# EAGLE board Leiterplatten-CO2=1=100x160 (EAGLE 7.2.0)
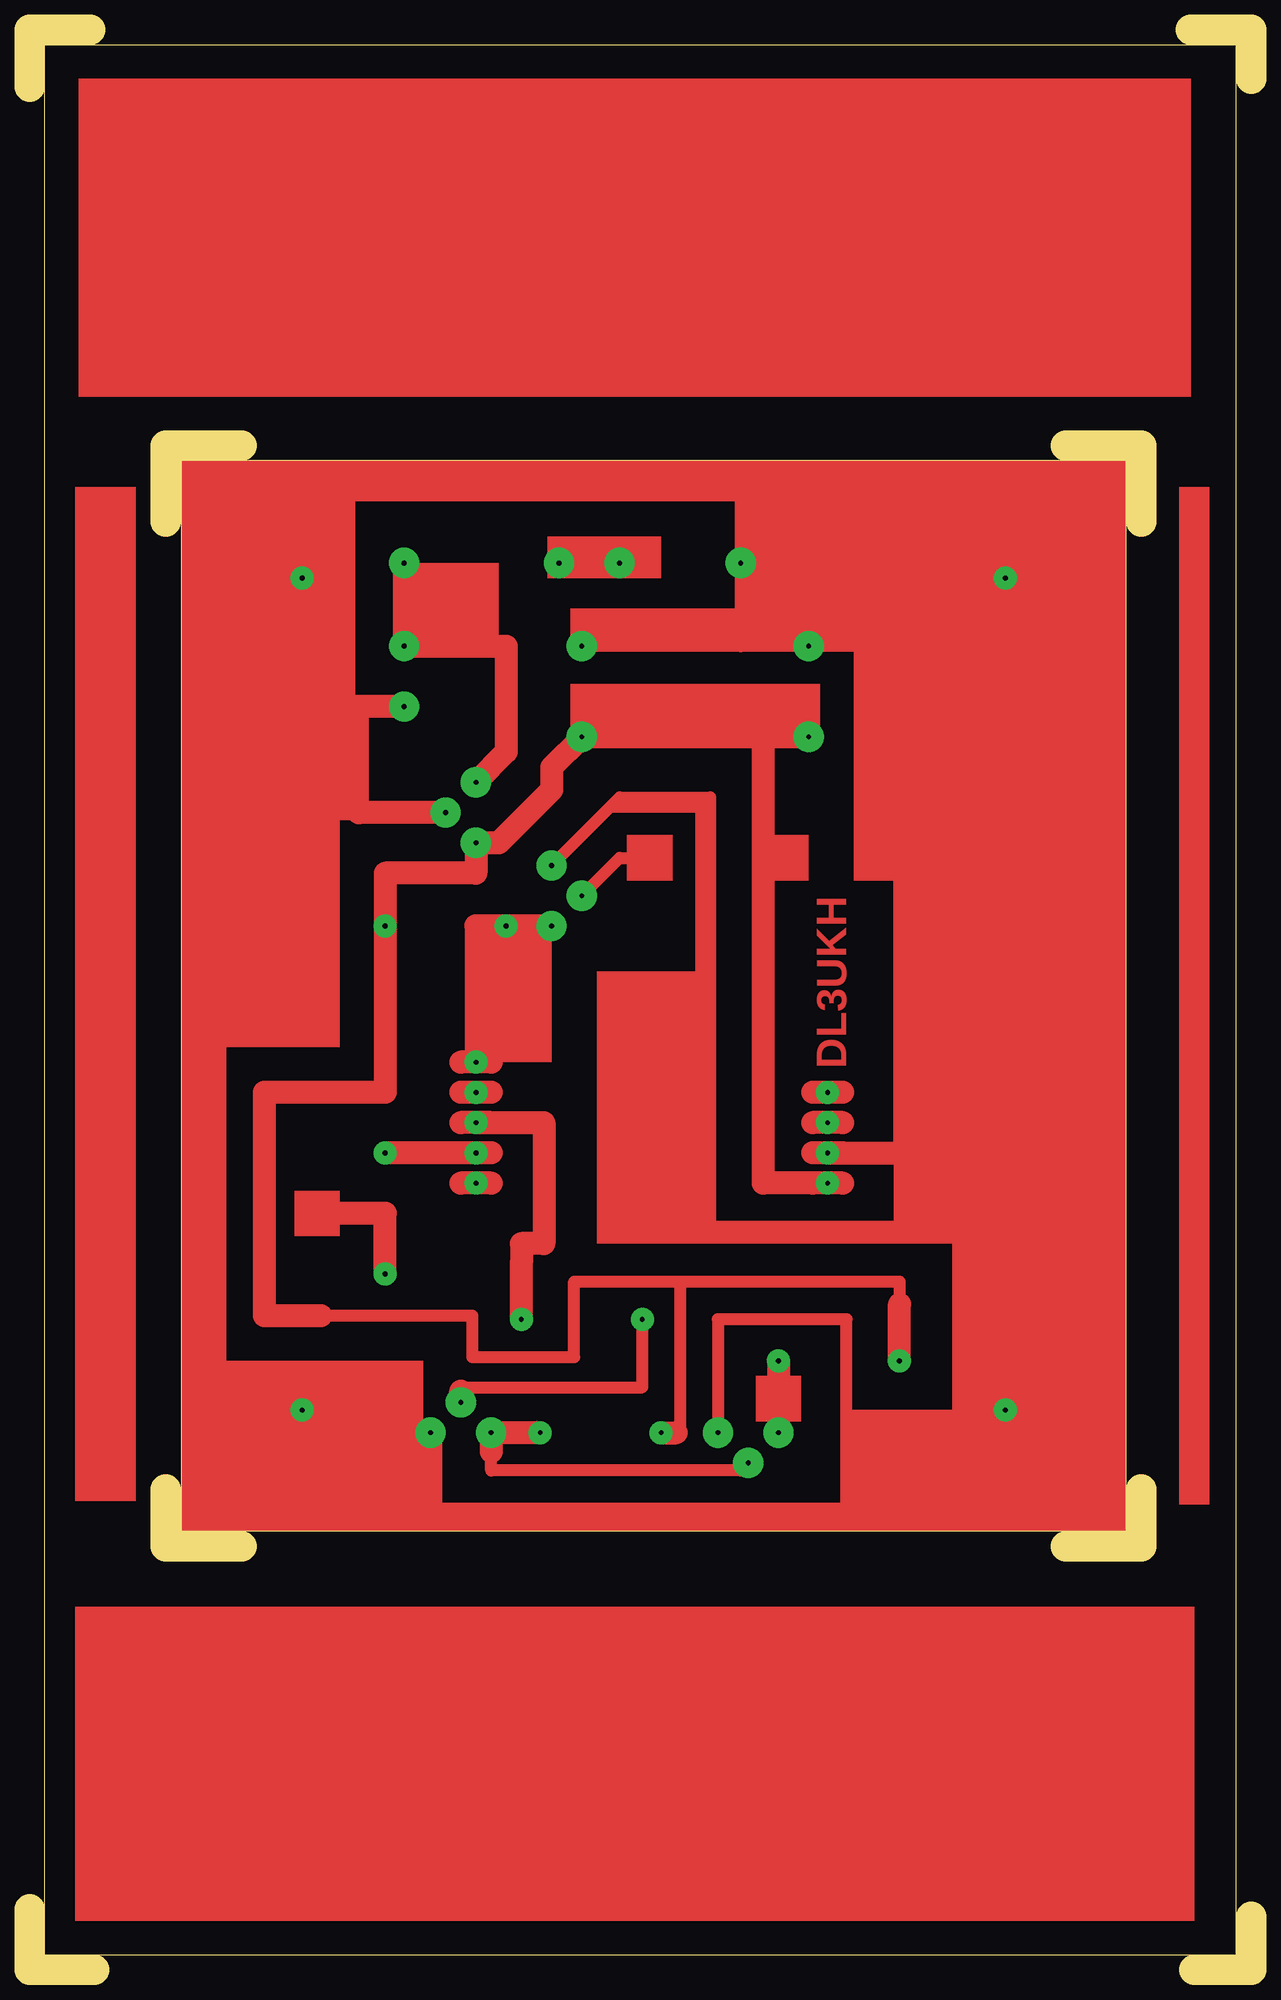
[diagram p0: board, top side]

Size 102.55 x 162.88 mm. Coordinates in mm from the lower left corner, seen from the top.
Outline: 5.4,0 0.32,0
Outline: 0,0 0,5.08
Outline: 97.79,0 102.55,0 102.55,4.45
Outline: 5.08,162.88 0,162.88 0,158.12
Outline: 102.55,158.75 102.55,162.88
Outline: 97.47,162.88 102.23,162.88
Outline: 11.43,121.6 11.43,127.95 17.78,127.95
Outline: 11.43,40.32 11.43,35.56 17.78,35.56
Outline: 86.99,35.56 93.34,35.56 93.34,40.32
Outline: 93.34,121.6 93.34,127.95 86.99,127.95
Outline: 1.27,1.27 101.28,1.27 101.28,161.61 1.27,161.61 1.27,1.27
Outline: 12.7,126.68 12.7,36.83 92.08,36.83 92.08,126.68 12.7,126.68
Copper layers (1*16): Top 0.035mm / dielectric 1.5mm / Bottom 0.035mm
Design rules "default": minimum track width 10mil, minimum drill 24mil, track to track 8mil, track to pad 8mil, pad to pad 8mil, via to via 8mil, smd to smd 8mil, copper to edge 40mil, drill to drill 8mil, minimum pad ring 10mil, minimum via ring 8mil, stop-mask expansion 4mil, vias tented up to drill 0mil, thermal gap 10mil

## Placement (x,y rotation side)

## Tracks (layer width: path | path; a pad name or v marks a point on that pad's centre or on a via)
S$1  (via drill 0.4 pad 1.93)
  Top 1.016: 37.47,71.12 37.15,71.12
  Top 1.93: 37.47,71.12 43.18,71.12 43.18,60.96 41.28,60.96 41.28,59.37 41.28,58.74 v41.28,54.61
S$2  (via drill 0.4 pad 1.93, 0.4 pad 2.54)
  Top 1.016: 24.45,54.93 37.15,54.93 37.15,51.44 45.72,51.44 45.72,57.79 54.61,57.79 | 54.29,45.09 54.61,45.09 54.61,57.79 | 54.61,57.79 73.02,57.79 73.02,55.88 | 29.84,92.08 v29.84,87.63 29.84,73.66
  Top 1.93: v65.41,103.5 61.6,103.5 | 61.6,103.5 v46.36,103.5 43.82,100.96 43.82,99.06 39.37,94.61 v37.47,94.61 37.47,92.08 29.84,92.08 29.84,73.66 19.68,73.66 19.68,54.93 24.45,54.93 | v66.99,66.04 61.6,66.04 61.6,103.5 | v73.02,51.12 73.02,55.88 | v53.02,45.09 54.29,45.09
S$3  (via drill 0.4 pad 2.54)
  Top 1.93: v49.53,118.11 v44.45,118.11
S$4  (via drill 0.4 pad 1.93)
  other vias: 37.47,73.66
S$5  (via drill 0.4 pad 2.54)
  Top 1.93: v31.43,118.11 v31.43,111.12 40.01,111.12 40.01,102.23 v37.47,99.69
S$6  (via drill 0.4 pad 1.93, 0.4 pad 2.54)
  Top 1.93: v62.87,51.12 v62.87,45.09
S$7  (via drill 0.4 pad 1.93)
  Top 1.93: v37.47,68.58 v29.84,68.58
S$8  (via drill 0.4 pad 1.93)
  other vias: 81.91,46.99
S$9  (via drill 0.4 pad 1.93)
  other vias: 81.91,116.84
S$10  (via drill 0.4 pad 1.93, 0.4 pad 2.54)
  Top 1.016: 73.02,68.58 73.02,61.6 | 73.34,68.58 80.64,68.58 80.64,111.12 73.02,111.12 | v31.43,106.05 27.94,106.05 | 27.94,106.05 27.94,97.16 34.61,97.16 v34.93,97.16 | 27.94,106.05 26.99,106.05 22.86,106.05 | 22.86,106.05 22.86,123.83 59.69,123.83 v59.69,118.11 59.69,111.12 | 59.69,111.12 v65.41,111.12 73.02,111.12 | 59.69,111.12 v46.36,111.12 | 22.86,106.05 14.92,106.05 14.92,38.74 33.66,38.74 | 33.66,38.74 33.66,39.05 | 33.66,38.74 68.58,38.74 68.58,54.61 57.79,54.61 v57.79,45.09 | 73.02,68.9 73.02,111.12
  Top 1.93: v66.99,68.58 73.02,68.58 73.34,68.58 | 34.61,97.16 27.62,97.16 | v31.43,106.05 26.99,106.05 | 33.66,39.05 v33.66,45.09 32.7,45.09
S$11  (via drill 0.4 pad 1.93)
  other vias: 37.47,66.04
S$12  (via drill 0.4 pad 1.93)
  Top 1.016: 25.4,63.5 23.5,63.5
  Top 1.93: v29.84,58.42 29.84,63.5 25.4,63.5
S$13
  Top 1.93: 68.26,73.66 65.72,73.66 | 68.26,71.12 65.72,71.12 | 38.74,73.66 36.2,73.66 | 38.74,76.2 36.2,76.2 | 38.74,66.04 36.2,66.04 | 38.74,68.58 36.2,68.58 | 68.26,68.58 65.72,68.58 | 38.74,71.12 36.2,71.12 | 68.26,66.04 65.72,66.04
S$14  (via drill 0.4 pad 1.93)
  other vias: 66.99,71.12
S$15  (via drill 0.4 pad 1.93)
  other vias: 66.99,73.66
S$16  (via drill 0.4 pad 1.93, 0.4 pad 2.54)
  Top 1.016: v60.33,42.55 59.69,41.91 38.74,41.91 38.74,43.5
  Top 1.93: v42.86,45.09 v38.74,45.09 38.74,43.5
S$17  (via drill 0.4 pad 1.93, 0.4 pad 2.54)
  Top 1.016: v43.82,87.63 v40.01,87.63 37.47,87.63
  Top 1.93: v43.82,87.63 37.47,87.63 v37.47,76.2
S$18  (via drill 0.4 pad 2.54)
  Top 1.016: v43.82,92.71 49.53,98.42 57.15,98.42 57.15,61.6
S$19  (via drill 0.4 pad 2.54)
  Top 1.016: v46.36,90.17 49.53,93.34 52.07,93.34
S$20  (via drill 0.4 pad 1.93, 0.4 pad 2.54)
  Top 1.016: 36.2,48.58 36.2,48.9 51.44,48.9 v51.44,54.61
  Top 1.93: v36.2,47.62 36.2,48.58
S$23  (via drill 0.4 pad 1.93)
  other vias: 37.47,71.12
S$29  (via drill 0.4 pad 1.93)
  other vias: 22.86,46.99
S$34  (via drill 0.4 pad 1.93)
  other vias: 22.86,116.84
(copper drawn outside any net)
  shapes: Top area x38

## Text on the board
Top: DL3UKH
